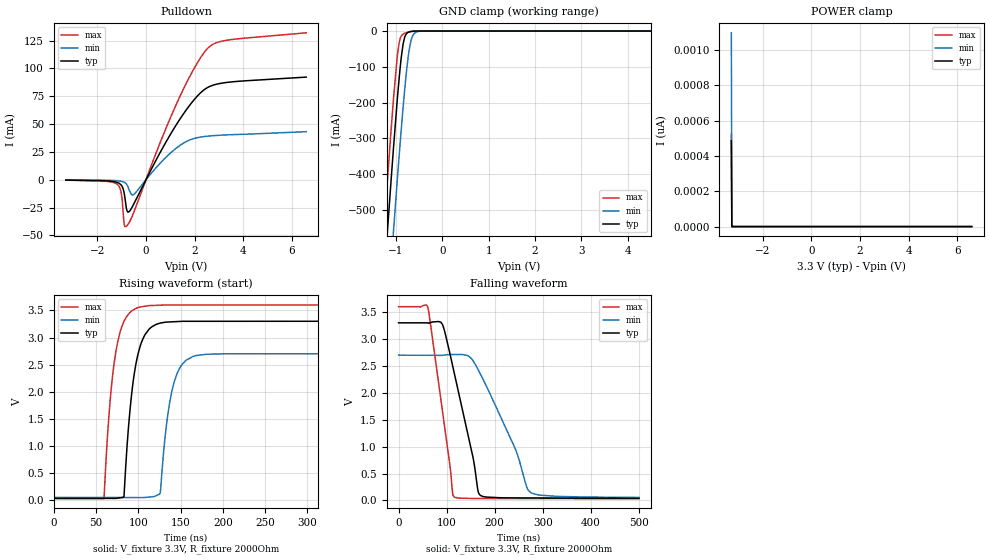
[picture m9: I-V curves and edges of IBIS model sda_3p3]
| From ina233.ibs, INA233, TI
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|   sda_3p3
[Model]   sda_3p3
Model_type   I/O_open_drain
Polarity   Non-Inverting
Vinl = 0.4
Vinh = 2.31
Vmeas = 1.65
Vref = 3.3
Cref = 2pF
Rref = 2000
|   typ   min   max
C_comp   1.203E-12   1.196E-12   1.271E-12
|C_comp_pull_down   1.360E-12   1.339E-12   1.374E-12
| Where Nom  PVT is Nominal Process, 3.3V, 25C
|   Fast PVT is Strong Process,  3.6V, -40C
|   Slow PVT is Weak Process,   2.7V, 125C
[Voltage Range]   3.3   2.7   3.6
[Temperature Range]   25   125   -40
[Pullup Reference]   3.3   2.7   3.6
[Pulldown Reference]   0   0   0
[Power Clamp Reference]   3.3   2.7   3.6
[GND Clamp Reference]   0   0   0
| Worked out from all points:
|   slope of the pulldown table from 0 to 0.495 V, typ, clamps not added: 23.7 ohm
|   GND clamp passes 1 mA (typ) near -0.67 V on its own axis
|   falling waveform, V_fixture 3.3V, R_fixture 2000Ohm: 20-80 % time 48.2ns typ, 75.8ns min, 32.9ns max; typ from 3.3 V to 0.039 V
|   rising waveform, V_fixture 3.3V, R_fixture 2000Ohm: 20-80 % time 13.6ns typ, 14ns min, 13.4ns max; typ from 0.039 V to 3.3 V
[Pulldown]
|   Voltage   I(typ)   I(min)   I(max)
-3.3V     -277.8uA   -132.7uA   -350.1uA
-1.191V   -2.338mA   -871.4uA   -3.896mA
-1.033V   -4.45mA    -1.339mA   -10.36mA
-983.4mV  -5.979mA   -1.591mA   -17.46mA
-894.3mV  -12.41mA   -2.333mA   -39.9mA
-815.1mV  -24.49mA   -3.669mA   -41.95mA
-745.8mV  -29.08mA   -6.081mA   -40.22mA
-508.2mV  -21.97mA   -13.35mA   -29.54mA
1.264V    49.95mA    28.7mA     68.48mA
2.511V    82.59mA    39.12mA    117.5mA
3.343V    87.49mA    40.35mA    125.4mA
6.6V      92.24mA    43.2mA     132mA
[GND Clamp]
|   Voltage   I(typ)   I(min)   I(max)
-3.3V     -4.686A    -4.907A    -4.556A
-1.29V    -760.6mA   -998mA     -618.3mA
-1.251V   -686.8mA   -924.1mA   -544.4mA
-1.181V   -559mA     -795.9mA   -417mA
-1.053V   -329.6mA   -562.7mA   -192.6mA
-973.5mV  -198.4mA   -424.1mA   -76.5mA
-924mV    -124.9mA   -340.5mA   -29.61mA
-815.1mV  -19.77mA   -171.5mA   -6.69mA
-735.9mV  -3.683mA   -74.37mA   -3.342mA
-676.5mV  -1.199mA   -28.91mA   -1.665mA
-508.2mV  -32.1uA    -958.7uA   -51.41uA
6.6V      0A         0A         0A
[POWER Clamp]
|   Voltage   I(typ)   I(min)   I(max)
-3.3V     486.6pA    1.097nA    522.5pA
-3.28V    0A         0A         0A
-3.27V    0A         0A         0A
6.6V      0A         0A         0A
[Ramp]
R_load = 2000
|   typ   min   max
dV/dt_r   1.95638/1.3574e-08   1.58677/1.40369e-08   2.14083/1.33924e-08
dV/dt_f   1.95638/4.81409e-08   1.58677/7.59945e-08   2.14083/3.29149e-08
[Falling Waveform]
V_fixture = 3.3V
V_fixture_min = 2.7V
V_fixture_max = 3.6V
R_fixture = 2000Ohm
C_fixture = 0F
|   Time   V(typ)   V(min)   V(max)
0s        3.3V       2.7V       3.6V
60.62ns   3.3V       2.697V     3.593V
91.07ns   3.273V     2.696V     1.672V
112.5ns   2.499V     2.711V     130.9mV
115.7ns   2.369V     2.711V     63.87mV
147ns     1.111V     2.672V     37.6mV
165.3ns   170.1mV    2.433V     34.96mV
170.2ns   93.49mV    2.348V     34.92mV
275ns     45.96mV    146.3mV    33.97mV
500ns     39.37mV    55.37mV    31.95mV
[Rising Waveform]
V_fixture = 3.3V
V_fixture_min = 2.7V
V_fixture_max = 3.6V
R_fixture = 2000Ohm
C_fixture = 0F
|   Time   V(typ)   V(min)   V(max)
0s        39.37mV    55.37mV    31.95mV
59.3ns    37.95mV    53.74mV    34.31mV
69.81ns   37.7mV     53.45mV    2.335V
82.87ns   60.97mV    53.09mV    3.291V
89.84ns   1.615V     52.9mV     3.456V
97.76ns   2.561V     52.68mV    3.54V
125.9ns   3.265V     140.7mV    3.595V
140.7ns   3.29V      2.082V     3.599V
164.3ns   3.298V     2.648V     3.599V
500ns     3.3V       2.7V       3.6V
